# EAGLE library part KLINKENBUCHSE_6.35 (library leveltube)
Klinkenbuchse für 6.35 mm Neutronik NEUTRIK NR-J6HF
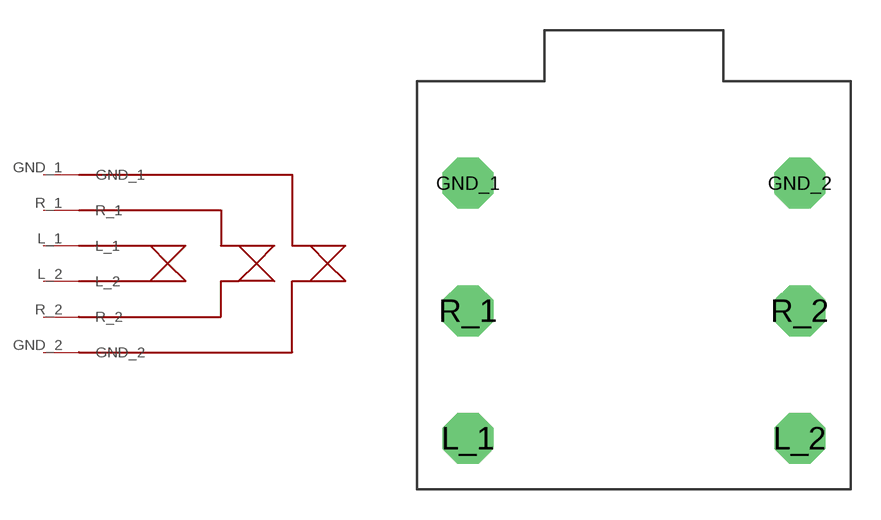
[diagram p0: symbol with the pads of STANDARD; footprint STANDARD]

Designator prefix -

## KLINKENBUCHSE_6.35  [STANDARD]
GND_1  GND_1
GND_2  GND_2
L_1  L_1
L_2  L_2
R_1  R_1
R_2  R_2

## Footprint STANDARD (pad centres in mm)
drill 1.3 pad 2.54 octagon: GND_1 2.54,15.24; GND_2 19.05,15.24; L_1 2.54,2.54; L_2 19.05,2.54; R_1 2.54,8.89; R_2 19.05,8.89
